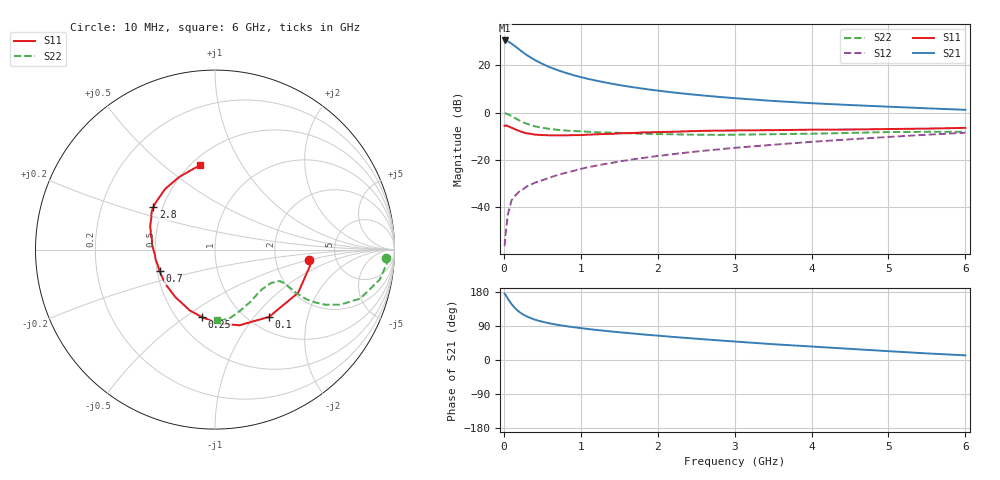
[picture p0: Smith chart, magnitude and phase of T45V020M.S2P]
! Infineon Technologies  Discrete & RF Semiconductors
! BFR182T
! Si NPN RF Bipolar Junction Transistor in SC75
! VCE = 5 V  IC = 20 mA
! Common Emitter S-Parameters:  October  1999
# GHz  S  MA  R  50
!  f  S11  S21  S12  S22
! GHz  MAG  ANG  MAG  ANG  MAG  ANG  MAG  ANG
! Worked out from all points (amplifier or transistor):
!   36 points, 10 MHz to 6 GHz, reference 50 ohm
!   highest |S21| = 30.6 dB at 10 MHz (marker M1)
!   |S21| within 3 dB of that: start of sweep to 167.6 MHz
!   unconditionally stable (mu >= 1): 706.5 MHz to 3.705 GHz
!   at 250 MHz: K = 0.64, MSG = 28.9 dB, |S12| = -32.4 dB
!   at 1.4 GHz: K = 1.10, MAG = 14.9 dB, |S12| = -21.3 dB
!   at 6 GHz: K = 0.85, MSG = 4.8 dB, |S12| = -8.5 dB
!   S11 on the Smith chart (normalised r, x): 10 MHz: 3.15, -0.52; 100 MHz: 1.22, -1.19; 250 MHz: 0.66, -0.58; 700 MHz: 0.52, -0.14; 2.8 GHz: 0.44, +0.25; 6 GHz: 0.55, +0.67
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0.01  0.5286 -6.5  33.73 175.0  0.0015 80.1  0.9564 -2.7
0.02  0.537 -9.7  33.69 172.7  0.0024 98.5  0.9641 -4.1
0.05  0.5219 -27.4  32.42 162.4  0.0068 83.5  0.9327 -10.3
0.1  0.4809 -51.2  28.93 147.7  0.014 72.2  0.8543 -18.6
0.15  0.4431 -72.2  25.14 135.7  0.0177 67.5  0.7629 -23.7
0.2  0.4109 -87.9  21.72 126.9  0.0214 66.6  0.6887 -26.5
0.25  0.383 -101.0  18.81 120.1  0.024 63.8  0.6272 -27.9
0.3  0.367 -112.5  16.48 114.7  0.0276 63.3  0.5817 -28.5
0.4  0.3447 -130.0  13.09 106.6  0.0328 63.8  0.5162 -28.2
0.5  0.3361 -142.0  10.8 101.0  0.0372 65.6  0.4789 -27.2
0.6  0.3321 -151.5  9.132 96.5  0.0425 67.0  0.4527 -26.6
0.7  0.3311 -158.9  7.933 92.8  0.0482 67.8  0.4335 -26.1
0.9  0.3355 -170.7  6.253 86.8  0.0584 70.0  0.4085 -25.9
1.1  0.3428 -179.7  5.175 81.6  0.0705 70.2  0.3944 -26.5
1.3  0.3537 173.5  4.42 77.2  0.0814 70.9  0.3818 -27.7
1.6  0.3705 165.2  3.617 71.3  0.0982 70.8  0.3679 -30.0
2.2  0.3945 154.2  2.682 60.9  0.1328 70.1  0.3492 -36.9
2.8  0.4171 145.4  2.155 51.7  0.1678 67.8  0.3394 -44.9
3.5  0.4267 135.8  1.771 41.7  0.2097 65.0  0.3503 -54.8
4.5  0.4405 123.7  1.452 29.4  0.2733 59.8  0.3731 -70.1
5.5  0.4605 107.8  1.238 17.4  0.3417 53.9  0.3942 -82.9
6  0.4772 100.1  1.15 12.3  0.3774 50.2  0.3941 -88.1
